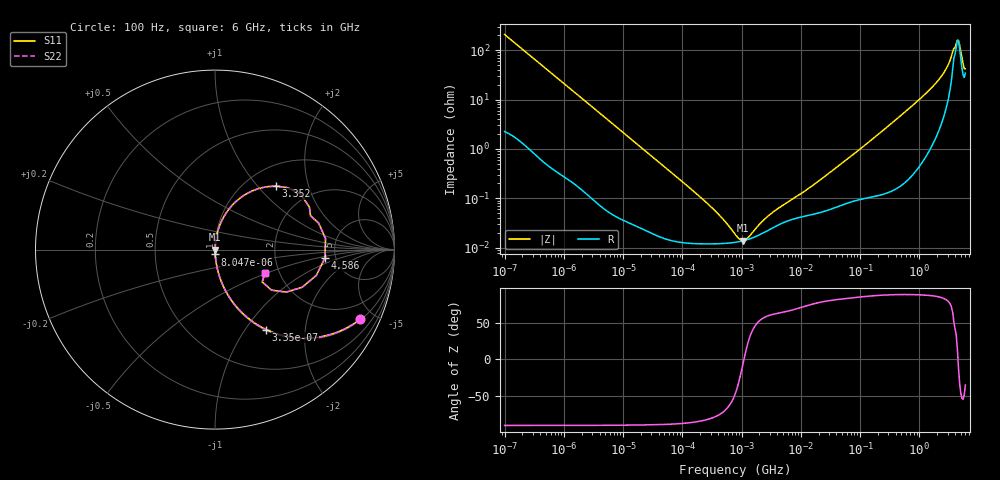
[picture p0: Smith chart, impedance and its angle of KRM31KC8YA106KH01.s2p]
!Murata Part Number: KRM31KC8YA106KH01
!These Parameters are Measured in Series Mode Connection
!Data Generated on Jan 08, 2026
!  o--ll--o
!Port1  Port2
!  o------o
!Operation Temp=25[degC], DC Bias Voltage=0[V]
!Freq. Start=100[Hz] Stop=6[GHz] 401[Steps]
# Hz S RI R 50
!Freq.(Hz) S11(Real) S11(Imag) S21(Real) S21(Imag) S12(Real) S12(Imag) S22(Real) S22(Imag)
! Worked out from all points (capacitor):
!   401 points, 100 Hz to 6 GHz, reference 50 ohm
!   read as one part in series: C = 7.62 uF near 109 Hz
!   lowest |Z| = 13.9 mohm at 1.06 MHz (marker M1)
!   series resonance near 1.095 MHz, so ESL is about 2.8 nH
!   S11 on the Smith chart (normalised r, x): 100 Hz: 1.04, -4.16; 335 Hz: 1.01, -1.26; 8.047 kHz: 1.00, -0.05; 3.352 GHz: 1.35, +1.26; 4.586 GHz: 4.09, -0.60; 6 GHz: 1.69, -0.48
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100  0.8098 -0.3871  0.1902 0.3871  0.1902 0.3871  0.8098 -0.3871
187  0.5553 -0.4907  0.4447 0.4907  0.4447 0.4907  0.5553 -0.4907
335  0.2854 -0.4457  0.7146 0.4457  0.7146 0.4457  0.2854 -0.4457
717  0.0828 -0.2696  0.9172 0.2696  0.9172 0.2696  0.0828 -0.2696
2008  0.0126 -0.1048  0.9874 0.1048  0.9874 0.1048  0.0126 -0.1048
8047  0.00113 -0.0267  0.9989 0.0267  0.9989 0.0267  0.00113 -0.0267
40335  0.000198 -0.00541  0.9998 0.00541  0.9998 0.00541  0.000198 -0.00541
302498  0.00012 -0.000669  0.9999 0.000669  0.9999 0.000669  0.00012 -0.000669
774597  0.000129 -0.000139  0.9999 0.000139  0.9999 0.000139  0.000129 -0.000139
1059725  0.000138 -1.26e-05  0.9999 1.26e-05  0.9999 1.26e-05  0.000138 -1.26e-05
1267578  0.000147 5.69e-05  0.9999 -5.69e-05  0.9999 -5.69e-05  0.000147 5.69e-05
3103719  0.00024 0.000421  0.9998 -0.000421  0.9998 -0.000421  0.00024 0.000421
1.555665e7  0.000473 0.00173  0.9995 -0.00173  0.9995 -0.00173  0.000473 0.00173
3.124326e8  0.00225 0.0303  0.9977 -0.0303  0.9977 -0.0303  0.00225 0.0303
9.150511e8  0.012 0.0899  0.988 -0.0899  0.988 -0.0899  0.012 0.0899
1.873145e9  0.0563 0.1952  0.9437 -0.1952  0.9437 -0.1952  0.0563 0.1952
2.679998e9  0.1532 0.2968  0.8468 -0.2968  0.8468 -0.2968  0.1532 0.2968
3.352442e9  0.3389 0.3541  0.6611 -0.3541  0.6611 -0.3541  0.3389 0.3541
4.009986e9  0.5324 0.1884  0.4676 -0.1884  0.4676 -0.1884  0.5324 0.1884
4.586474e9  0.6128 -0.0457  0.3872 0.0457  0.3872 0.0457  0.6128 -0.0457
5.245841e9  0.3964 -0.2369  0.6036 0.2369  0.6036 0.2369  0.3964 -0.2369
6e9  0.2789 -0.128  0.7211 0.128  0.7211 0.128  0.2789 -0.128
